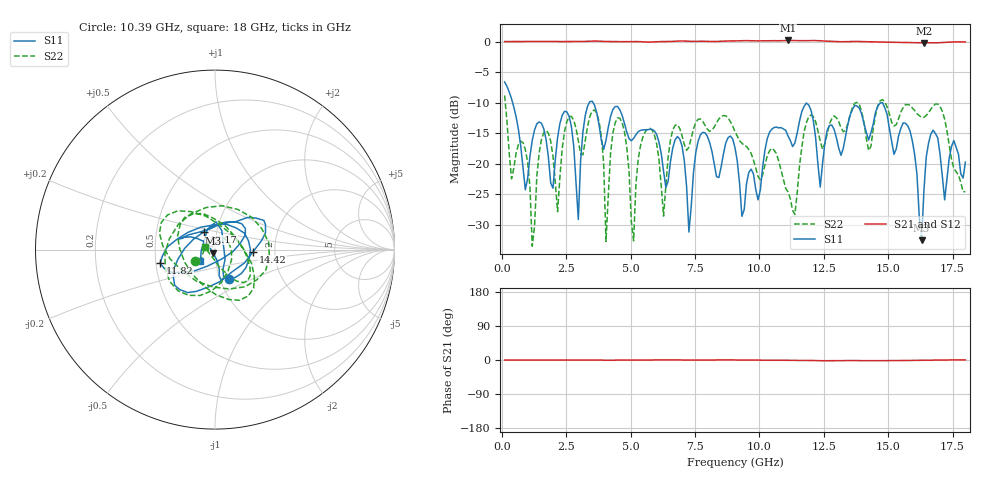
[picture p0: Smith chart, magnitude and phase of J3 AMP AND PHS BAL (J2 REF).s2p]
!Agilent Technologies,E8364B,MY43040528,A.07.50.67
!Agilent E8364B: A.07.50.67
!Date: Wednesday, May 04, 2022 12:47:33
!Correction: S11(Full 2 Port(1,2))
!S21(Full 2 Port(1,2))
!S12(Full 2 Port(1,2))
!S22(Full 2 Port(1,2))
!S2P File: Measurements: S11, S21, S12, S22:
# Hz S  dB  R 50
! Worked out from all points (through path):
!   201 points, 100 MHz to 18 GHz, reference 50 ohm
!   highest |S21| = 0.19 dB at 11.11 GHz (marker M1); lowest = -0.2 dB at 16.39 GHz (marker M2)
!   lowest |S11| = -32.5 dB at 16.3 GHz (marker M3), VSWR 1.05, Z = 48.8 - j2 ohm
!   |S11| at or under -10 dB: 411.1 MHz to 3.39 GHz (2.979 GHz wide, 157 % of centre); 3.536 GHz to 14.76 GHz (11.22 GHz wide, 123 % of centre); 14.78 GHz to end of sweep
!   |S22| runs from -33.5 to -8.8 dB; largest |S21 - S12| = 0.02
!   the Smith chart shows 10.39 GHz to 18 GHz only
!   S11 on the Smith chart (normalised r, x): 10.39 GHz: 1.11, -0.37; 11.82 GHz: 0.53, -0.09; 13.17 GHz: 0.87, +0.18; 14.42 GHz: 1.54, -0.04; 18 GHz: 0.84, -0.11
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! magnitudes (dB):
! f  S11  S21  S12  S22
! 100 MHz  -6.6  0.0  0.1  -8.8
! 1.174 GHz  -16.1  0.0  0.1  -33.5
! 1.621 GHz  -14.3  0.0  0.1  -14.9
! 2.964 GHz  -29.1  0.0  0.1  -16.2
! 3.143 GHz  -14.7  0.0  0.1  -18.5
! 3.769 GHz  -13.6  0.1  0.1  -13.1
! 4.038 GHz  -16.2  0.0  0.1  -32.7
! 4.486 GHz  -10.6  0.0  0.1  -12.5
! 5.112 GHz  -15.8  0.0  0.1  -32.6
! 6.096 GHz  -16.5  0.0  0.1  -19.3
! 7.26 GHz  -31.2  0.1  0.1  -17.3
! 9.05 GHz  -17.4  0.1  0.2  -14.7
! 10.39 GHz  -14.8  0.2  0.2  -17.9
! 11.11 GHz  -15.4  0.2  0.2  -24.6
! 11.82 GHz  -10.1  0.2  0.2  -13.3
! 12.09 GHz  -12.9  0.2  0.3  -12.3
! 13.17 GHz  -18.6  0.0  0.0  -14.1
! 14.42 GHz  -13.5  0.0  0.0  -14.2
! 15.05 GHz  -14.2  -0.1  0.0  -11.8
! 16.3 GHz  -32.5  -0.2  -0.1  -12.4
! 16.39 GHz  -24.4  -0.2  -0.1  -12.4
! 18 GHz  -19.7  0.0  0.0  -24.6
